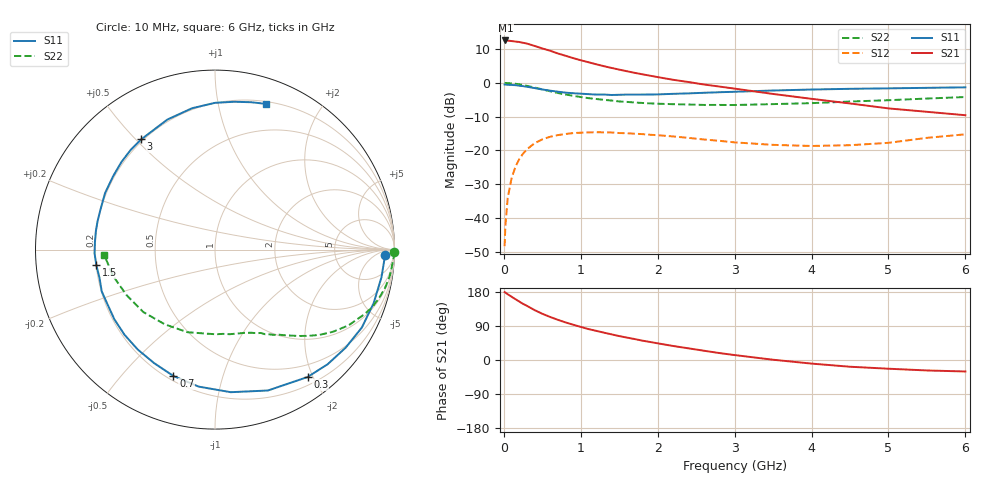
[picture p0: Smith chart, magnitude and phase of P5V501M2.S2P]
! SIEMENS Small Signal Semiconductors
! BFP183
! Si NPN RF Bipolar Junction Transistor in SOT143
! VCE = 0.5 V  IC = 1.2 mA
! Common Emitter S-Parameters:  March  1996
# GHz  S  MA  R  50
!  f  S11  S21  S12  S22
! GHz  MAG  ANG  MAG  ANG  MAG  ANG  MAG  ANG
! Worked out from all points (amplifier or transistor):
!   36 points, 10 MHz to 6 GHz, reference 50 ohm
!   highest |S21| = 12.6 dB at 20 MHz (marker M1)
!   |S21| within 3 dB of that: start of sweep to 595.4 MHz
!   unconditionally stable (mu >= 1): 2.185 GHz to end of sweep
!   at 250 MHz: K = 0.12, MSG = 16.4 dB, |S12| = -21.0 dB
!   at 1.4 GHz: K = 0.64, MSG = 9.6 dB, |S12| = -14.7 dB
!   at 6 GHz: K = 1.37, MAG = -0.8 dB, |S12| = -15.2 dB
!   S11 on the Smith chart (normalised r, x): 10 MHz: 29, -16; 300 MHz: 0.31, -1.92; 700 MHz: 0.22, -0.70; 1.5 GHz: 0.20, -0.06; 3 GHz: 0.19, +0.52; 6 GHz: 0.22, +1.39
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0.01  0.9481 -1.7  4.255 179.1  0.0038 86.8  0.998 -0.8
0.02  0.9444 -3.9  4.261 178.0  0.0076 85.2  0.9986 -1.7
0.05  0.9403 -9.4  4.243 173.5  0.0196 85.7  0.9925 -4.2
0.1  0.933 -18.6  4.176 167.1  0.0385 78.2  0.9849 -8.5
0.2  0.9102 -36.9  4.042 154.3  0.074 67.9  0.9532 -16.5
0.25  0.8954 -45.5  3.936 148.1  0.0894 62.5  0.9308 -20.4
0.3  0.8775 -54.0  3.832 142.9  0.1037 57.9  0.905 -23.6
0.4  0.8386 -69.4  3.535 131.6  0.1276 48.9  0.8551 -29.6
0.5  0.7993 -83.7  3.242 122.0  0.1456 41.3  0.8016 -34.8
0.6  0.7687 -96.8  3.006 113.7  0.1589 34.5  0.7527 -39.1
0.7  0.7413 -108.2  2.738 106.2  0.1682 28.7  0.71 -42.6
0.8  0.7177 -118.2  2.532 99.3  0.1747 23.7  0.6735 -45.6
0.9  0.7038 -127.7  2.335 93.2  0.1804 19.3  0.6442 -48.1
1.1  0.682 -145.3  2.027 81.6  0.1847 11.6  0.5949 -52.9
1.5  0.6668 -172.5  1.575 63.1  0.1807 0.3  0.5306 -61.1
1.8  0.672 170.8  1.343 51.1  0.1743 -5.3  0.5045 -66.6
2.2  0.6888 152.8  1.113 37.0  0.161 -11.3  0.4839 -75.2
3  0.7392 123.8  0.823 13.0  0.1314 -14.6  0.4705 -95.0
3.5  0.7717 110.1  0.686 0.7  0.1207 -10.7  0.4851 -108.4
4.5  0.8177 90.0  0.496 -17.8  0.1193 2.2  0.5299 -139.0
5.5  0.8455 76.2  0.373 -27.6  0.1534 9.8  0.5867 -165.5
6  0.8606 70.6  0.332 -30.3  0.1729 8.1  0.618 -177.3
